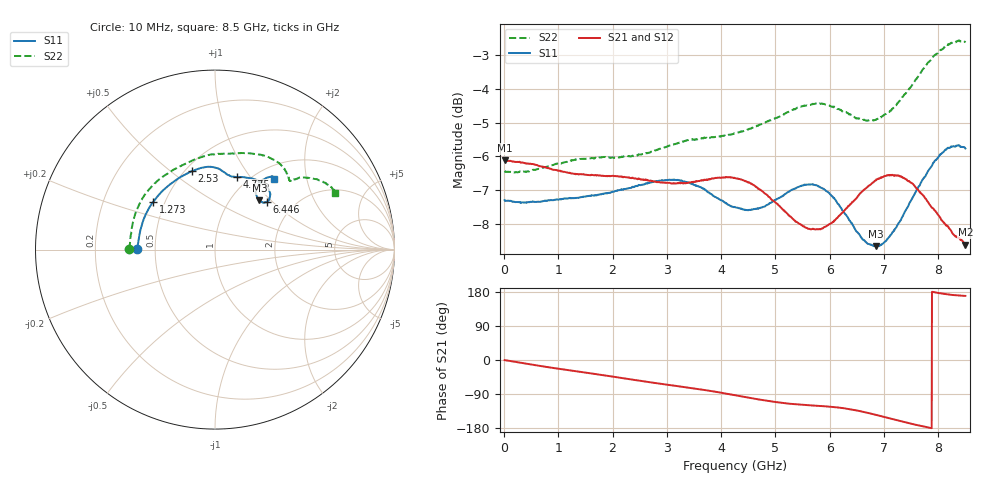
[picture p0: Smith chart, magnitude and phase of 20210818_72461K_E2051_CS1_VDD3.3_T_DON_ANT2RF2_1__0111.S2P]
!Agilent Technologies,E5071C,MY46417908,A.11.23
!Date: Wed Aug 18 14:28:00 2021
!Data & Calibration Information:
!Freq	S11:SOLT2(ON)	S21:SOLT2(ON)	S12:SOLT2(ON)	S22:SOLT2(ON)
!PortZ  Port1:50+j0  Port2:50+j0
!Above PortZ is port z conversion or system Z0 setting when saving the data.
!When reading, reference impedance value at option line is always used.
# Hz S dB R 50
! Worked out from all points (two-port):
!   1601 points, 10 MHz to 8.5 GHz, reference 50 ohm
!   highest |S21| = -6.11 dB at 10 MHz (marker M1); lowest = -8.6 dB at 8.5 GHz (marker M2)
!   |S21| within 3 dB of the highest: start of sweep to end of sweep
!   lowest |S11| = -8.6 dB at 6.85 GHz (marker M3), VSWR 2.17, Z = 67.3 + j42.8 ohm
!   |S11| at or under -10 dB: nowhere
!   |S22| runs from -6.5 to -2.6 dB; largest |S21 - S12| = 0.0018
!   S11 on the Smith chart (normalised r, x): 10 MHz: 0.40, +0.00; 1.273 GHz: 0.43, +0.28; 2.53 GHz: 0.54, +0.60; 4.775 GHz: 0.88, +0.87; 6.446 GHz: 1.47, +0.93; 8.5 GHz: 1.21, +1.31
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1e7  -7.29 179.6  -6.11 -0.4  -6.11 -0.4  -6.43 179.6
7.369562e8  -7.31 159.4  -6.31 -17.3  -6.31 -17.3  -6.33 160.3
1.272888e9  -7.23 142.3  -6.51 -28.6  -6.51 -28.6  -6.11 144.5
1.426769e9  -7.20 137.1  -6.52 -31.8  -6.53 -31.7  -6.07 140.0
2.026375e9  -7.04 118.6  -6.58 -44.4  -6.59 -44.4  -6.04 122.8
2.530469e9  -6.84 106.4  -6.68 -55.3  -6.68 -55.3  -5.94 110.2
2.843538e9  -6.72 100.2  -6.75 -61.9  -6.75 -62.0  -5.79 103.4
3.406e9  -6.77 90.6  -6.77 -73.2  -6.76 -73.2  -5.51 92.7
3.910094e9  -7.21 83.7  -6.64 -84.2  -6.63 -84.2  -5.42 85.0
4.255e9  -7.50 79.7  -6.64 -92.9  -6.63 -92.9  -5.31 80.6
4.775012e9  -7.49 73.2  -7.05 -106.0  -7.04 -106.0  -5.02 73.5
5.289719e9  -6.99 62.3  -7.79 -115.9  -7.80 -115.8  -4.64 64.4
5.671769e9  -6.83 53.1  -8.14 -120.0  -8.15 -120.0  -4.46 56.8
6.048512e9  -7.18 45.3  -7.94 -123.8  -7.96 -123.9  -4.53 49.7
6.446481e9  -8.09 42.7  -7.31 -131.7  -7.31 -131.9  -4.82 44.5
6.658731e9  -8.51 44.4  -6.95 -138.1  -6.95 -138.1  -4.93 42.8
6.849756e9  -8.65 47.9  -6.71 -144.7  -6.72 -144.7  -4.92 42.3
7.088538e9  -8.39 52.8  -6.55 -153.4  -6.57 -153.4  -4.69 41.8
7.497119e9  -7.31 56.8  -6.78 -168.0  -6.78 -168.1  -3.95 39.3
7.868556e9  -6.30 54.8  -7.48 -179.6  -7.46 -179.7  -3.15 33.8
8.20285e9  -5.75 52.0  -8.12 172.6  -8.11 172.7  -2.69 28.5
8.5e9  -5.76 50.2  -8.60 169.1  -8.57 169.2  -2.64 25.2
